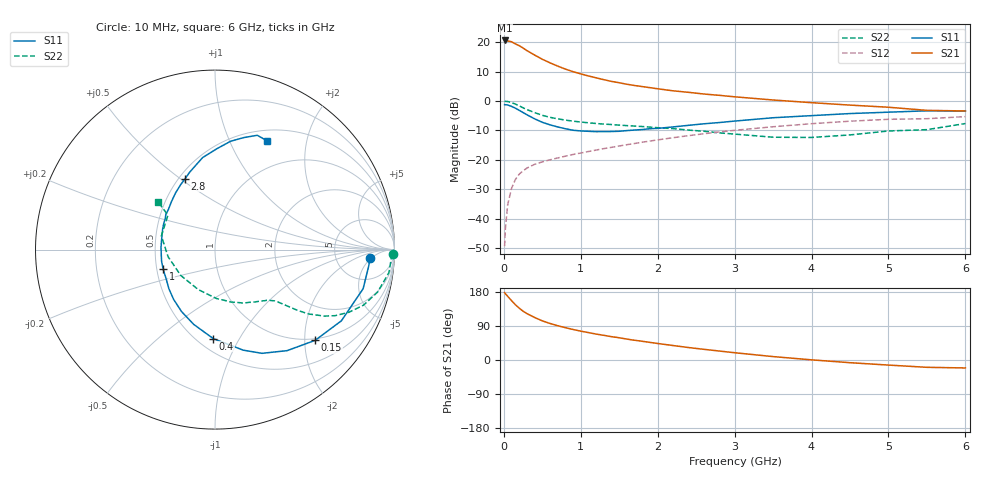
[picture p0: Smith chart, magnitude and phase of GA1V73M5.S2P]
! Infineon Technologies  Discrete & RF Semiconductors
! BF775
! Si NPN RF Bipolar Junction Transistor in SOT23
! VCE = 1.75 V  IC = 3.5 mA
! Common Emitter S-Parameters:  May  1996
# GHz  S  MA  R  50
!  f  S11  S21  S12  S22
! GHz  MAG  ANG  MAG  ANG  MAG  ANG  MAG  ANG
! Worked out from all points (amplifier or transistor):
!   36 points, 10 MHz to 6 GHz, reference 50 ohm
!   highest |S21| = 20.6 dB at 10 MHz (marker M1)
!   |S21| within 3 dB of that: start of sweep to 274.3 MHz
!   unconditionally stable (mu >= 1): 881.8 MHz to 4.317 GHz; 5.165 GHz to end of sweep
!   at 250 MHz: K = 0.40, MSG = 20.9 dB, |S12| = -23.7 dB
!   at 1.4 GHz: K = 1.15, MAG = 8.8 dB, |S12| = -15.8 dB
!   at 6 GHz: K = 1.01, MAG = 0.4 dB, |S12| = -5.3 dB
!   S11 on the Smith chart (normalised r, x): 10 MHz: 12, -4; 150 MHz: 0.96, -2.24; 400 MHz: 0.60, -0.78; 1 GHz: 0.54, -0.13; 2.8 GHz: 0.54, +0.52; 6 GHz: 0.63, +1.39
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0.01  0.8647 -3.0  10.66 177.8  0.0034 86.4  0.9933 -1.5
0.02  0.8617 -5.9  10.51 175.0  0.0067 87.7  0.9835 -3.0
0.05  0.8536 -14.8  10.47 168.1  0.0172 81.4  0.9771 -7.6
0.1  0.8082 -29.4  10.12 156.7  0.0326 74.4  0.9367 -14.6
0.15  0.7529 -42.2  9.318 145.8  0.0462 67.5  0.8836 -20.5
0.2  0.6915 -54.5  8.689 136.9  0.0569 62.3  0.8248 -25.0
0.25  0.6346 -65.6  7.923 128.8  0.065 58.3  0.764 -28.8
0.3  0.582 -74.3  7.163 122.5  0.0722 55.7  0.7133 -31.3
0.4  0.496 -91.1  6.019 112.2  0.0837 51.8  0.6331 -34.5
0.5  0.4332 -105.9  5.106 103.3  0.0921 50.0  0.5695 -36.4
0.6  0.3923 -118.4  4.438 96.4  0.0999 49.4  0.5265 -37.5
0.7  0.361 -129.6  3.908 90.5  0.1073 49.2  0.4956 -38.4
0.8  0.337 -139.7  3.473 85.3  0.115 49.0  0.4724 -39.2
1  0.3088 -159.5  2.88 76.2  0.1301 49.8  0.4378 -40.7
1.1  0.3046 -167.7  2.657 72.3  0.1381 50.2  0.4247 -42.0
1.6  0.3131 158.7  1.918 55.1  0.1803 50.0  0.3806 -49.0
2.2  0.3614 132.1  1.484 38.2  0.2369 47.4  0.3386 -61.7
2.8  0.429 112.8  1.245 23.7  0.297 42.5  0.2865 -80.0
3.5  0.5177 97.6  1.037 9.0  0.364 34.5  0.2416 -112.6
4.5  0.6099 81.8  0.849 -7.1  0.4527 21.6  0.2643 -171.4
5.5  0.6791 69.7  0.691 -19.3  0.4987 7.0  0.3249 143.8
6  0.672 64.6  0.675 -21.0  0.541 2.9  0.4125 140.1
